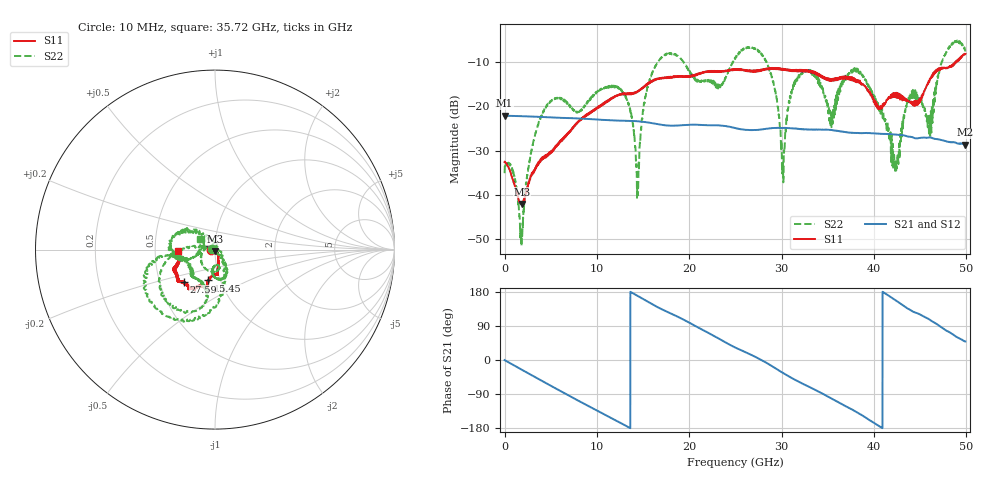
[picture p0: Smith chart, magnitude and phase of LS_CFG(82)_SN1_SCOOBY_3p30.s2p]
!Keysight Technologies,N5245B,MY58422026,A.13.80.08
!Date: Thursday, March 19, 2020 23:52:45
!Correction: S11(Full 2 Port(1,2))
!S21(Full 2 Port(1,2))
!S12(Full 2 Port(1,2))
!S22(Full 2 Port(1,2))
!S2P File: Measurements: S11, S21, S12, S22:
# Hz S DB R 50.0
!freq dBS11 angS11 dBS21 angS21 dBS12 angS12 dBS22 angS22
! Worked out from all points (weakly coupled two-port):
!   4991 points, 10 MHz to 49.91 GHz, reference 50 ohm
!   highest |S21| = -22.07 dB at 10 MHz (marker M1); lowest = -28.6 dB at 49.91 GHz (marker M2)
!   lowest |S11| = -42.0 dB at 1.9 GHz (marker M3), VSWR 1.02, Z = 49.8 - j0.763 ohm
!   |S11| at or under -10 dB: start of sweep to 48.78 GHz; 48.81199 GHz to 48.87663 GHz (64.64 MHz wide, 0.132 % of centre)
!   |S22| runs from -51.5 to -5.1 dB; largest |S21 - S12| = 0.00077
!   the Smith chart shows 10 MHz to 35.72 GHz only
!   S11 on the Smith chart (normalised r, x): 10 MHz: 0.95, -0.01; 15.45 GHz: 0.87, -0.31; 27.59 GHz: 0.67, -0.25; 35.72 GHz: 0.66, -0.02
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1e7  -32.56 -173.1  -22.07 -0.3  -22.06 -0.3  -35.06 176.6
1.9e9  -42.05 -104.2  -22.19 -26.1  -22.18 -26.0  -49.42 15.6
4.23e9  -31.79 -54.3  -22.39 -57.5  -22.39 -57.4  -21.04 -151.0
8.33e9  -22.96 -74.2  -22.75 -112.0  -22.74 -111.9  -20.76 -91.4
1.266e10  -17.32 -83.6  -23.22 -167.4  -23.21 -167.3  -16.40 -66.7
1.44e10  -16.53 -95.9  -23.34 169.3  -23.33 169.4  -37.50 -118.6
1.545e10  -15.07 -102.8  -23.60 154.5  -23.59 154.6  -15.78 176.0
1.665e10  -13.79 -102.2  -24.02 138.6  -24.01 138.7  -9.84 -158.0
2.496e10  -11.73 -124.4  -24.84 33.2  -24.83 33.4  -9.24 -168.2
2.759e10  -12.06 -134.2  -25.24 3.1  -25.24 3.3  -7.72 -109.5
2.92e10  -11.37 -140.4  -24.87 -19.8  -24.87 -19.5  -15.47 -71.7
3.014e10  -11.65 -143.5  -24.88 -33.7  -24.88 -33.4  -33.18 28.5
3.125e10  -11.77 -148.6  -24.96 -49.4  -24.96 -49.0  -15.35 137.7
3.328e10  -12.15 -156.9  -25.21 -74.6  -25.21 -74.2  -12.24 -174.0
3.572e10  -13.71 -176.6  -25.44 -105.9  -25.37 -105.4  -20.11 149.5
3.816e10  -14.52 172.5  -26.01 -137.9  -25.96 -138.0  -11.41 -174.7
4.16e10  -17.95 103.9  -26.24 169.7  -26.26 169.7  -25.43 71.4
4.245e10  -17.15 101.8  -26.36 156.0  -26.38 156.0  -33.92 -172.5
4.39e10  -18.95 74.0  -26.84 132.5  -26.85 132.7  -17.59 -32.8
4.601e10  -14.38 8.9  -26.98 106.9  -27.00 107.0  -23.08 115.7
4.771e10  -11.29 5.9  -27.79 79.6  -27.81 79.8  -8.19 -79.7
4.991e10  -8.15 -14.7  -28.62 48.9  -28.65 49.0  -7.33 -14.8
